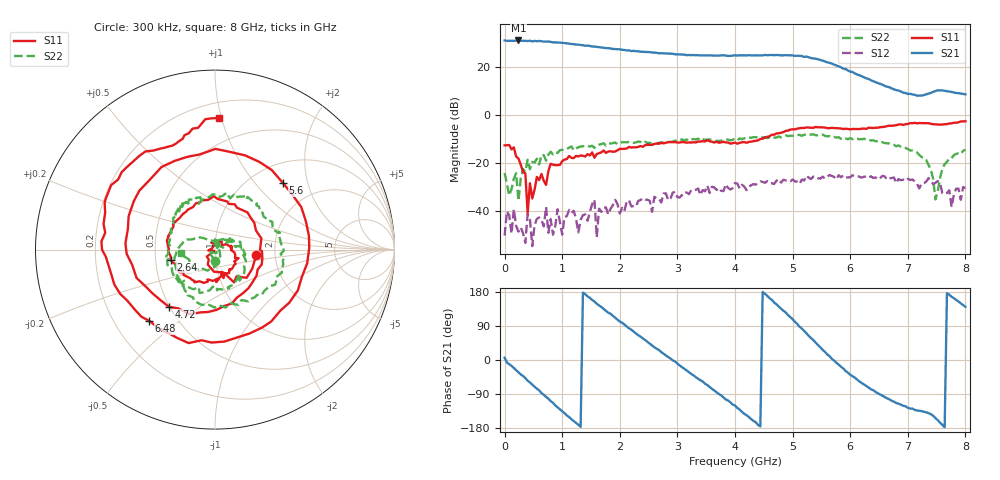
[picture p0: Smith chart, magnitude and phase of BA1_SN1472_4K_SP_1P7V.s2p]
! VC=1.7V IC=9.25mA
# HZ S DB R 50.00
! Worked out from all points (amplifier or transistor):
!   201 points, 300 kHz to 8 GHz, reference 50 ohm
!   highest |S21| = 30.9 dB at 240.3 MHz (marker M1)
!   |S21| within 3 dB of that: start of sweep to 1.713 GHz
!   unconditionally stable (mu >= 1): start of sweep to 3.505 GHz; 3.531 GHz to 3.823 GHz; 6.064 GHz to end of sweep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
!   at 1.32 GHz: K = 2.59, MAG = 29.4 dB, |S12| = -43.7 dB
!   at 4 GHz: K = 0.90, MSG = 26.6 dB, |S12| = -28.4 dB
!   at 8 GHz: K = 2.74, MAG = 12.3 dB, |S12| = -30.5 dB
!   S11 on the Smith chart (normalised r, x): 300 kHz: 1.60, -0.10; 2.64 GHz: 0.60, -0.07; 4.72 GHz: 0.49, -0.38; 5.6 GHz: 1.38, +1.42; 6.48 GHz: 0.35, -0.39; 8 GHz: 0.31, +0.98
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300000  -12.68 -7.1  30.90 6.1  -50.20 30.9  -24.21 -89.7
4.02985e7  -12.64 -27.4  30.77 -6.7  -40.11 54.7  -28.61 -163.3
2.40291e8  -18.16 -92.6  30.91 -32.2  -48.55 148.1  -35.64 32.0
5.202805e8  -31.14 96.6  30.73 -70.4  -45.85 172.8  -19.84 24.5
7.602715e8  -23.39 26.6  30.47 -102.0  -49.00 72.4  -16.52 7.3
1.08026e9  -18.39 -22.9  29.72 -146.1  -42.11 63.5  -14.15 -32.5
1.360249e9  -17.02 -55.3  28.94 177.7  -41.67 26.4  -13.08 -71.1
1.640238e9  -15.93 -81.6  28.10 143.9  -39.02 2.2  -12.40 -102.7
2.000225e9  -14.14 -109.2  27.21 101.6  -40.98 -44.0  -11.85 -139.8
2.640201e9  -11.95 -167.3  25.78 29.7  -34.90 -84.1  -11.82 167.6
2.6802e9  -12.02 -172.0  25.56 26.4  -34.91 -83.2  -11.64 165.8
3.360174e9  -11.09 112.5  24.77 -49.4  -30.62 -126.5  -9.90 120.5
4.00015e9  -11.50 13.7  24.75 -120.3  -28.37 166.0  -9.80 78.6
4.400135e9  -10.61 -65.9  24.70 -171.3  -28.26 136.3  -9.27 50.2
4.720123e9  -7.76 -129.0  24.88 147.1  -27.41 112.9  -9.46 29.2
5.08011e9  -5.75 158.8  24.57 95.3  -27.81 75.1  -8.37 2.0
5.360099e9  -5.40 99.2  23.45 52.5  -25.69 48.4  -8.10 -19.2
5.60009e9  -5.51 44.3  21.81 14.8  -25.80 20.7  -8.92 -40.0
5.920078e9  -5.77 -26.2  19.06 -28.9  -25.99 -6.4  -9.79 -70.2
6.480057e9  -5.35 -132.7  13.19 -87.9  -26.86 -61.4  -10.90 -125.7
6.68005e9  -4.53 -160.9  11.44 -103.9  -26.39 -86.3  -11.90 -147.0
8e9  -2.69 88.4  8.51 140.3  -30.47 -176.7  -14.48 -174.9
